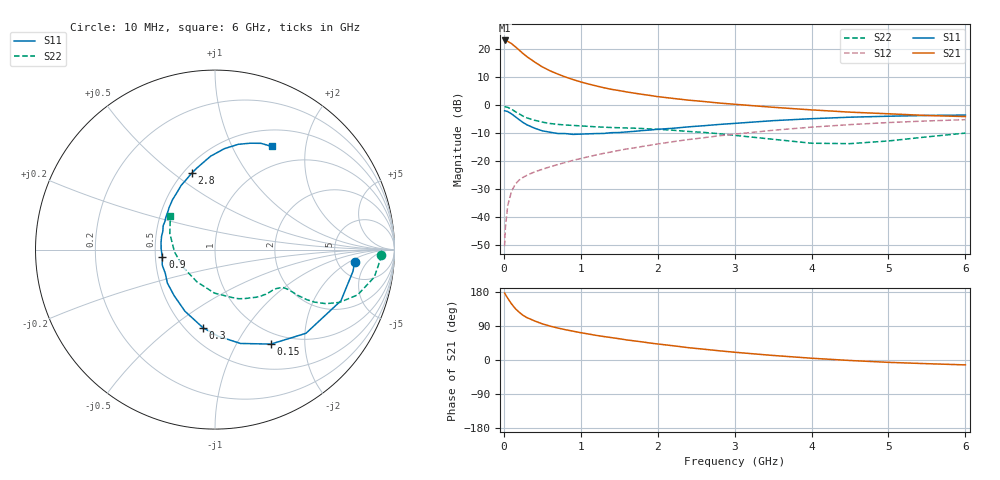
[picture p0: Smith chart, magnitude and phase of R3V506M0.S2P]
! SIEMENS Small Signal Semiconductors
! BFR181
! Si NPN RF Bipolar Junction Transistor in SOT23
! VCE = 0.5 V  IC = 6 mA
! Common Emitter S-Parameters:  May  1996
# GHz  S  MA  R  50
!  f  S11  S21  S12  S22
! GHz  MAG  ANG  MAG  ANG  MAG  ANG  MAG  ANG
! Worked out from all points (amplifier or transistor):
!   36 points, 10 MHz to 6 GHz, reference 50 ohm
!   highest |S21| = 23.0 dB at 10 MHz (marker M1)
!   |S21| within 3 dB of that: start of sweep to 181 MHz
!   unconditionally stable (mu >= 1): 460.3 MHz to end of sweep
!   at 250 MHz: K = 0.67, MSG = 22.1 dB, |S12| = -25.9 dB
!   at 1.4 GHz: K = 1.41, MAG = 7.4 dB, |S12| = -16.8 dB
!   at 6 GHz: K = 1.12, MAG = -1.5 dB, |S12| = -5.3 dB
!   S11 on the Smith chart (normalised r, x): 10 MHz: 7.28, -2.50; 150 MHz: 0.83, -1.40; 300 MHz: 0.61, -0.65; 900 MHz: 0.54, -0.05; 2.8 GHz: 0.55, +0.59; 6 GHz: 0.71, +1.44
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0.01  0.7814 -4.9  14.06 176.6  0.003 88.6  0.9278 -1.9
0.02  0.7783 -8.9  13.88 173.0  0.0064 82.3  0.92 -4.1
0.05  0.7573 -22.1  13.56 163.2  0.0158 78.0  0.9007 -9.8
0.1  0.6887 -42.6  12.35 148.0  0.0287 69.0  0.8341 -17.6
0.15  0.6116 -59.4  10.83 135.4  0.0385 61.7  0.7532 -23.0
0.2  0.5419 -74.8  9.456 126.0  0.0455 57.8  0.687 -26.0
0.25  0.4827 -88.0  8.197 117.8  0.0507 55.0  0.6269 -27.8
0.3  0.4396 -98.9  7.228 111.9  0.0553 53.7  0.5833 -28.6
0.4  0.382 -116.0  5.803 103.1  0.0635 53.4  0.5292 -28.9
0.5  0.3432 -131.5  4.749 95.4  0.0706 54.0  0.4909 -28.7
0.6  0.3243 -144.9  4.048 89.5  0.0782 54.7  0.4637 -28.6
0.7  0.307 -154.4  3.541 84.4  0.0856 55.9  0.4473 -28.8
0.9  0.2963 -171.7  2.819 76.0  0.1021 57.4  0.4287 -29.6
1.1  0.3031 172.7  2.349 68.6  0.1184 58.3  0.4122 -31.5
1.3  0.3081 160.7  2.015 61.9  0.1361 58.5  0.3992 -33.7
1.6  0.3286 146.3  1.691 52.9  0.1632 58.1  0.3854 -38.0
2.2  0.3812 124.0  1.3 37.6  0.2197 55.1  0.3513 -49.1
2.8  0.446 106.8  1.074 24.3  0.2799 50.3  0.3044 -64.1
3.5  0.5209 92.7  0.903 12.0  0.351 42.8  0.2425 -90.7
4.5  0.6009 77.5  0.739 -1.3  0.443 29.7  0.2026 -150.0
5.5  0.6451 66.6  0.644 -9.7  0.5149 16.3  0.2677 160.2
6  0.6557 61.3  0.616 -12.9  0.5421 9.4  0.3123 142.7
